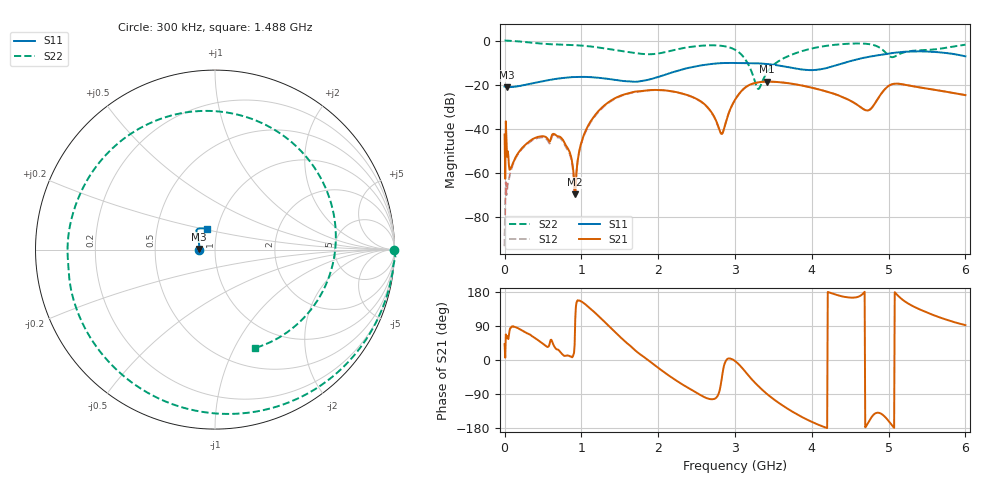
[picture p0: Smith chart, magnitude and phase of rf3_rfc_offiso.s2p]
!Agilent Technologies,M9375A,MY55441453,A.02.50.04
!Agilent M9375A: A.02.50.04
!Date: Monday, December 12, 2016 11:34:39
!Correction: S11(Full 2 Port(1,2))
!S21(Full 2 Port(1,2))
!S12(Full 2 Port(1,2))
!S22(Full 2 Port(1,2))
!S2P File: Measurements: S11, S21, S12, S22:
# Hz S  dB  R 50
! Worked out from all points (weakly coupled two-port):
!   751 points, 300 kHz to 6 GHz, reference 50 ohm
!   highest |S21| = -18.61 dB at 3.416 GHz (marker M1); lowest = -69.7 dB at 920.3 MHz (marker M2)
!   lowest |S11| = -21.1 dB at 32.3 MHz (marker M3), VSWR 1.19, Z = 41.9 + j0.293 ohm
!   |S11| at or under -10 dB: start of sweep to 4.43 GHz
!   |S22| runs from -21.9 to 0.1 dB; largest |S21 - S12| = 0.014
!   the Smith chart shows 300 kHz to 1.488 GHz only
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300000  -20.82 -177.2  -42.57 41.8  -93.16 26.3  -0.03 -0.2
3.22984e7  -21.12 177.7  -52.60 63.5  -67.83 90.6  -0.04 -9.7
8.0296e7  -21.07 172.0  -57.91 84.8  -59.13 94.3  -0.13 -23.7
3.042848e8  -19.81 152.8  -46.25 69.7  -46.62 69.0  -0.79 -89.8
6.40268e8  -17.50 138.9  -42.28 38.4  -42.78 38.9  -1.71 177.0
8.322584e8  -16.67 135.2  -49.42 11.6  -50.08 12.8  -1.94 129.7
9.20254e8  -16.51 133.2  -69.69 108.6  -68.63 120.1  -2.09 108.1
1.00025e9  -16.46 131.2  -46.17 154.5  -46.41 155.4  -2.28 87.5
1.264237e9  -17.01 122.9  -30.45 108.1  -30.81 109.7  -3.35 8.6
1.520224e9  -18.26 107.8  -24.84 58.0  -25.02 59.6  -4.73 -78.3
1.768212e9  -18.41 81.3  -22.93 14.6  -23.02 16.2  -5.98 -159.4
2.0002e9  -16.49 55.0  -22.38 -20.7  -22.43 -19.7  -5.86 123.5
2.448178e9  -11.99 32.7  -25.58 -80.7  -25.68 -80.3  -2.74 24.5
2.824159e9  -10.22 28.6  -42.27 -53.6  -42.35 -51.5  -2.38 -31.8
3.00015e9  -10.16 28.7  -26.83 -2.7  -26.91 -2.2  -4.15 -70.1
3.296135e9  -10.31 29.5  -18.97 -67.3  -18.99 -66.6  -21.77 133.7
3.416129e9  -10.63 27.5  -18.61 -89.6  -18.61 -89.0  -14.45 24.3
4.0001e9  -13.40 -14.6  -21.34 -163.2  -21.35 -163.0  -3.58 -102.7
4.720064e9  -7.51 -64.4  -31.68 -170.4  -31.69 -170.0  -1.50 -155.9
5.00005e9  -5.91 -62.9  -20.56 -160.9  -20.57 -160.7  -6.82 -172.4
5.232038e9  -5.03 -61.3  -20.15 151.8  -20.14 152.0  -5.05 -161.4
6e9  -7.14 -58.0  -24.71 91.9  -24.71 92.0  -1.87 99.2
